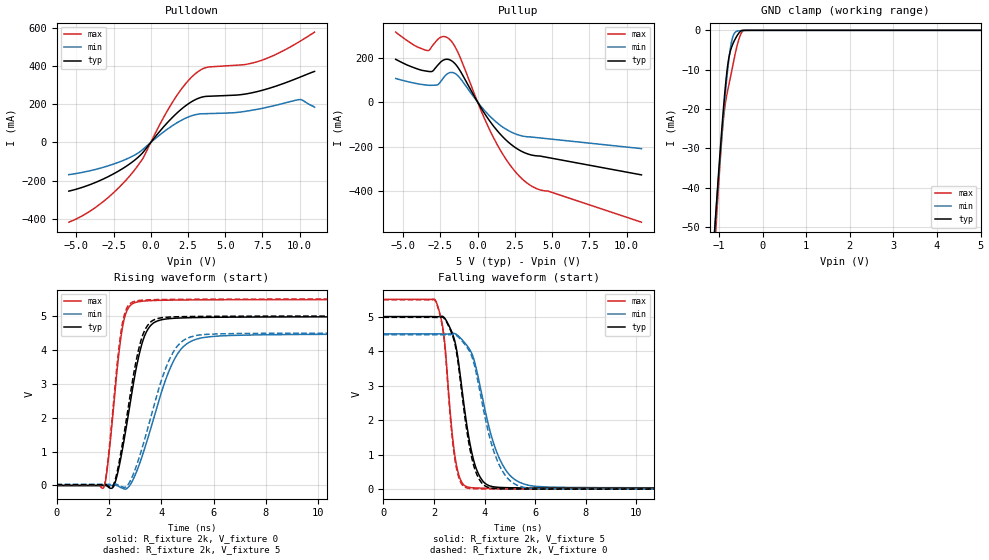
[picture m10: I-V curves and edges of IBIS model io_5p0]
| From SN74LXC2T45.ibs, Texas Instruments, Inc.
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[Model]   io_5p0
Model_type  I/O
Vinl=1.35
Vinh=3.85
Enable   Active-Low
Vref =   0
Rref =   2000
Cref =   15p
Vmeas =   2.5
| variable   typ   min   max
C_comp   5.79pF   4.92pF   7.16pF
| C_pullup   14.63pF   5.87pF   28.02pF
| C_pulldown   8.69pF   6.31pF   14.42pF
| C_tri-state   5.79pF   4.92pF   7.16pF
[Temperature Range]   40   100   -40
| Ambient temperature   25   85   -40
[Voltage range]   5   4.5   5.5
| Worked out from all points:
|   slope of the pulldown table from 0 to 0.75 V, typ, clamps not added: 10.5 ohm
|   slope of the pullup table from 0 to 0.75 V, typ, clamps not added: 9.47 ohm
|   GND clamp passes 1 mA (typ) near -0.56 V on its own axis
|   rising waveform, R_fixture 2k, V_fixture 0: 20-80 % time 693ps typ, 1.13ns min, 437ps max; typ from 0 V to 4.98 V
|   falling waveform, R_fixture 2k, V_fixture 5: 20-80 % time 605ps typ, 928ps min, 399ps max; typ from 5 V to 0.025 V
|   rising waveform, R_fixture 2k, V_fixture 5: 20-80 % time 665ps typ, 1.05ns min, 425ps max; typ from 0.025 V to 5 V
|   falling waveform, R_fixture 2k, V_fixture 0: 20-80 % time 581ps typ, 863ps min, 389ps max; typ from 4.98 V to 0 V
[GND Clamp]
| LXC8T245_IO_50
|   Voltage   I(typ)   I(min)   I(max)
-5.5V     -897.1mA   -831.9mA   -1.015A
-1.115V   -53.49mA   -53.1mA    -58.66mA
-1.08V    -47.7mA    -47.75mA   -52.14mA
-1.05V    -42.82mA   -43.24mA   -46.67mA
-915mV    -22.23mA   -23.93mA   -24.75mA
-870mV    -16.24mA   -18.06mA   -19.86mA
-810mV    -9.725mA   -11mA      -15.84mA
-710mV    -4.241mA   -2.794mA   -10.43mA
-595mV    -1.535mA   -238.1uA   -4.333mA
-495mV    -143.9uA   -74.43uA   -859.9uA
-410mV    -2.841uA   -26.45uA   -7.398uA
5V        42.75pA    201.5nA    680.2pA
[Pulldown]
| LXC8T245_IO_50
|   Voltage   I(typ)   I(min)   I(max)
-5.5V     -253.8mA   -167.8mA   -415.9mA
-3.43V    -199.2mA   -134.9mA   -323mA
-1.42V    -112.1mA   -79.11mA   -175.4mA
-515mV    -51.25mA   -34.88mA   -81.44mA
675mV     64.66mA    43.62mA    103.8mA
1.605V    142.3mA    95.28mA    227.8mA
2.375V    193.6mA    128.1mA    310mA
3.085V    226.9mA    146.6mA    364.6mA
3.83V     241.1mA    150.7mA    393.4mA
7.4V      270.6mA    177.1mA    427.6mA
10.03V    341.2mA    224.3mA    528.3mA
11V       371.1mA    184.2mA    576.2mA
[Pullup]
| LXC8T245_IO_50
|   Voltage   I(typ)   I(min)   I(max)
-5.5V     192.6mA    106.5mA    315.1mA
-3.39V    139mA      76.44mA    232.1mA
-3.02V    139.4mA    75.83mA    254.6mA
-2.445V   182.3mA    95.48mA    292.9mA
-1.78V    187.3mA    133.5mA    275.4mA
-1.265V   150.4mA    114.7mA    215.4mA
270mV     -30.29mA   -22.56mA   -44.29mA
1.205V    -119.5mA   -87.17mA   -177.6mA
2.245V    -190.4mA   -134.4mA   -289.3mA
3.285V    -231.3mA   -155.7mA   -362.5mA
4.095V    -242.4mA   -160.5mA   -392.8mA
11V       -327.5mA   -209.3mA   -540.4mA
[Ramp]
| LXC8T245_IO_50
| variable   typ   min   max
dV/dt_r   3.0/7.18E-10   2.7/7.02E-10   3.3/7.15E-10
dV/dt_f   3.0/4.5E-10   2.7/6.34E-10   3.3/4.41E-10
R_load = 2k
[Rising Waveform]
| LXC8T245_IO_50
R_fixture =   2k
C_fixture =   0
L_fixture =   0
V_fixture =   0
V_fixture_min = 0
V_fixture_max = 0
|   Time   V(typ)   V(min)   V(max)
0s        447.4pV    5.606nV    1.8nV
1.82ns    4.313mV    -101.6uV   -36.37mV
2.185ns   -21.19mV   8.283mV    2.348V
2.52ns    1.074V     -82.14mV   4.664V
2.735ns   2.048V     -55.44mV   5.226V
3.075ns   3.572V     440.1mV    5.412V
3.555ns   4.681V     1.565V     5.452V
4.435ns   4.93V      3.617V     5.47V
5.525ns   4.957V     4.353V     5.477V
29.99ns   4.978V     4.473V     5.483V
[Falling Waveform]
| LXC8T245_IO_50
R_fixture =   2k
C_fixture =   0
L_fixture =   0
V_fixture =   5
V_fixture_min = 4.5
V_fixture_max = 5.5
|   Time   V(typ)   V(min)   V(max)
0s        5V         4.5V       5.5V
2.085ns   4.997V     4.5V       5.43V
2.385ns   4.985V     4.497V     4.498V
2.69ns    4.579V     4.508V     1.836V
2.865ns   4.152V     4.492V     791.6mV
3.35ns    1.619V     4.116V     58.61mV
3.815ns   362.5mV    3.013V     31.48mV
4.56ns    53.14mV    933.4mV    24.28mV
5.735ns   34.84mV    113.1mV    21.05mV
29.99ns   24.92mV    33.45mV    17.03mV
[Rising Waveform]
| LXC8T245_IO_50
R_fixture =   2k
C_fixture =   0
L_fixture =   0
V_fixture =   5
V_fixture_min = 4.5
V_fixture_max = 5.5
|   Time   V(typ)   V(min)   V(max)
0s        24.84mV    32.98mV    17.02mV
1.81ns    28.89mV    32.9mV     -26.1mV
2.175ns   17.26mV    40.3mV     2.42V
2.5ns     1.151V     -37.61mV   4.71V
2.705ns   2.125V     -1.781mV   5.262V
3.025ns   3.609V     520mV      5.443V
3.475ns   4.717V     1.658V     5.477V
4.295ns   4.968V     3.685V     5.489V
5.335ns   4.987V     4.426V     5.495V
29.99ns   5V         4.5V       5.5V
[Falling Waveform]
| LXC8T245_IO_50
R_fixture =   2k
C_fixture =   0
L_fixture =   0
V_fixture =   0
V_fixture_min = 0
V_fixture_max = 0
|   Time   V(typ)   V(min)   V(max)
0s        4.979V     4.474V     5.484V
2.085ns   4.975V     4.475V     5.412V
2.385ns   4.962V     4.471V     4.444V
2.68ns    4.556V     4.481V     1.794V
2.85ns    4.133V     4.47V      755.3mV
3.32ns    1.591V     4.096V     30.82mV
3.765ns   318.2mV    3.021V     7.91mV
4.48ns    14.77mV    869.1mV    3.507mV
5.555ns   3.694mV    51.86mV    1.999mV
29.99ns   75.9uV     271.6uV    10.25uV
